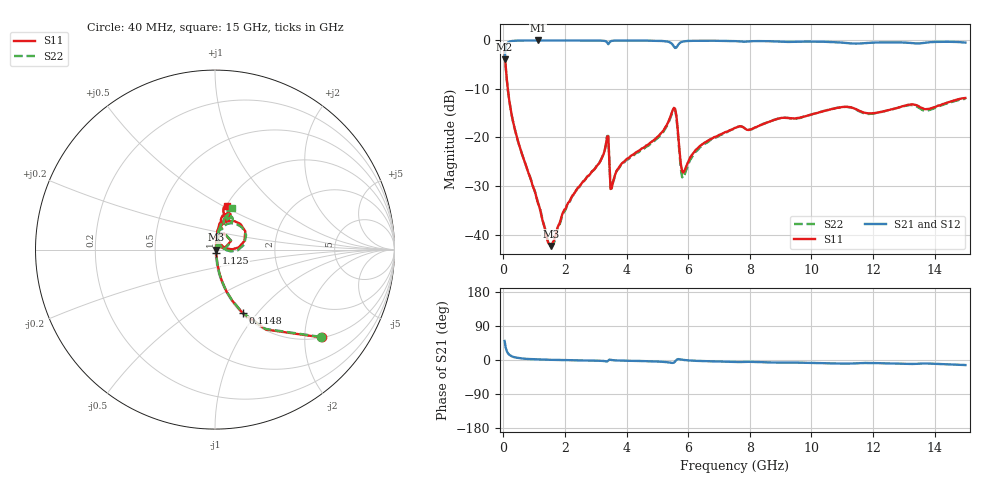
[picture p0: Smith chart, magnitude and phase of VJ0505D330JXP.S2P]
! VJ0505D330JXP
! MLCC placed on 25 mil thick microstrip substrate in series configuraton.
! DATE 06/29/2018  09:16
! CORRECTED  DATA
# GHz  S  MA  R  50.00
!  FREQ  S11M  S11A  S21M  S21A  S12M  S12A  S22M  S22A
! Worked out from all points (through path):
!   401 points, 40 MHz to 15 GHz, reference 50 ohm
!   highest |S21| = -0.08 dB at 1.125 GHz (marker M1); lowest = -3.9 dB at 40 MHz (marker M2)
!   group delay of S21, straight-line fit = 3.07 ps
!   lowest |S11| = -42.3 dB at 1.536 GHz (marker M3), VSWR 1.02, Z = 50.8 - j0.0295 ohm
!   |S11| at or under -10 dB: 143.8 MHz to end of sweep
!   |S22| runs from -42.3 to -2.3 dB; largest |S21 - S12| = 0.0026
!   S11 on the Smith chart (normalised r, x): 40 MHz: 1.01, -2.42; 114.8 MHz: 1.01, -0.84; 1.125 GHz: 1.01, -0.04; 15 GHz: 1.00, +0.53
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0.04  0.7696 -39.5  0.6347 50.1  0.6353 50.2  0.763 -39.6
0.1148  0.385 -66.5  0.9152 22.6  0.9161 22.7  0.3816 -66.6
0.1896  0.2433 -74.5  0.9615 14.1  0.9622 14.1  0.2414 -74.6
0.3766  0.1198 -79.8  0.984 6.9  0.9845 7.0  0.1192 -79.9
1.1246  0.0211 -68.3  0.9908 1.5  0.9911 1.6  0.02139 -69.9
1.536  0.007691 -2.2  0.9906 0.5  0.9908 0.6  0.007673 -7.4
2.0222  0.01859 66.1  0.9908 -0.2  0.9905 -0.2  0.01819 65.3
2.5458  0.03411 76.9  0.9891 -1.0  0.9897 -0.9  0.03413 74.7
3.1068  0.05428 79.3  0.987 -2.0  0.9876 -1.9  0.05418 77.2
3.3312  0.08547 70.8  0.9694 -3.5  0.97 -3.4  0.08651 68.4
3.5556  0.0345 68.7  0.9845 -0.5  0.9849 -0.5  0.03409 66.6
3.8922  0.05553 80.8  0.9884 -1.7  0.9888 -1.7  0.05447 78.9
5.0516  0.1045 81.5  0.9813 -4.2  0.9818 -4.1  0.1012 77.8
5.5378  0.2013 45.3  0.8579 -6.8  0.8585 -6.7  0.1948 39.6
5.6126  0.1705 16.1  0.8349 -0.4  0.8356 -0.3  0.1649 9.6
5.7622  0.05309 14.5  0.9482 1.4  0.949 1.5  0.04766 7.0
5.8744  0.04526 53.2  0.971 -0.0  0.9715 0.0  0.04038 50.5
6.3232  0.07829 80.3  0.9837 -2.4  0.9847 -2.3  0.07509 78.1
7.52  0.1254 79.8  0.9755 -5.1  0.9763 -5.1  0.125 77.0
10.0258  0.173 78.8  0.9642 -7.8  0.9657 -7.8  0.1731 73.3
12.5316  0.1913 73.0  0.9488 -9.1  0.9497 -9.1  0.1908 69.6
15  0.2542 75.0  0.9426 -13.3  0.943 -13.4  0.2492 67.8
